(*
xml 存n行，每行4个参数，bool-可用位vaild、bool-输出位状态、bool-正反向输出标记位、lreal-节点坐标
*)

FUNCTION_BLOCK FB_EL5131_MultiCycle
VAR CONSTANT
	{attribute 'displaymode':='hex'}
	cMaxCounterValue										: 	UDINT := 4294967295;
	{attribute 'hide'}
	cMaxNumOfOutputPreCycle									:	USINT := 8;	 
END_VAR
VAR_INPUT
	{attribute 'hide'} // 隐藏该变量
	nDistWindow												:	UINT := 5;// pulse
	stEl5131												:	REFERENCE TO ST_EL5131;
	bReset													:	BOOL;
	bExecute												:	BOOL;
	bSetRefPos												:	BOOL;
	rRefPos													:	LREAL; // 以参考轴位置(mm)进行初始化
	rScaleFactor      										: 	LREAL := 1; // 分子/分母		            						: 	BYTE := 2#1111_1111;
	{attribute 'displaymode':='bin'}
	OutputOption											:	BYTE := 2#0000_0001; // chn 1 output
	InputOption												:	ST_EL5131_Setting;
	pstEL5131_CamData										:	POINTER TO ST_EL5131_CamData;
	nSize													:	ULINT;
	cNum													:	UDINT;// 点总数 >0
END_VAR
VAR_IN_OUT
	nActNum													:	UDINT;// presistent 第 0 个开始
END_VAR
VAR_OUTPUT
	bBusy													:	BOOL;
	bDone													:	BOOL;
	bError													:	BOOL;
	nErrId													:	UDINT;
	{attribute 'hide'}
	sErr													:	STRING;
END_VAR
VAR
	{attribute 'hide'}
	{attribute 'displaymode':='hex'}
	tDCTIME64												:	ULINT;
	{attribute 'hide'}
	{attribute 'displaymode':='hex'}
	LastTimeStampsOutChn1X64								: 	ARRAY[1..8] OF ULINT;
	{attribute 'hide'}
	{attribute 'displaymode':='hex'}
	LastTimeStampsOutChn2X64								: 	ARRAY[1..8] OF ULINT;
	{attribute 'hide'}
	_pLastTimeStampsOutChnX64								:	POINTER TO ARRAY[1..8] OF ULINT;
	{attribute 'hide'}
	{attribute 'displaymode':='hex'}
	TimeStampsOutChn1X64									: 	ARRAY[1..8] OF ULINT;
	{attribute 'hide'}
	{attribute 'displaymode':='hex'}
	TimeStampsOutChn2X64									: 	ARRAY[1..8] OF ULINT;
	{attribute 'hide'}
	{attribute 'displaymode':='hex'}
	_pTimestampChnX64										:	POINTER TO ARRAY[1..8] OF ULINT;// Point to stEl5131.PdoToPlc
	{attribute 'hide'}
	{attribute 'displaymode':='hex'}
	pPdoTimestampChnX32										:	POINTER TO ARRAY[1..8] OF ULINT;// Point to stEl5131.PdoToPlc
	{attribute 'hide'}
	rtReset                 								: 	R_TRIG;
	{attribute 'hide'}
	rtExecute                 								: 	R_TRIG;
	{attribute 'hide'}
	rtSetRefPos                								: 	R_TRIG;
	{attribute 'hide'}
	{attribute 'displaymode':='bin'}
	_nMem													:	WORD;// bit 0=reset ,bit 1=READY_TEMP load  
	{attribute 'hide'}
	_pControl												:	POINTER TO ST_Control_UINT_TO_BIT;
	{attribute 'hide'}
	_pControOutput											:	POINTER TO ST_ENC_Control_Output_Channel;
	{attribute 'hide'}
	i														:	INT;
	{attribute 'hide'}
	j														:	UDINT;
	eState													:	(INIT,LOAD,READY,RUN,FINISH);
	{attribute 'hide'}
	_tSetParDelay100ms										:	TON :=(PT:= T#0MS);
	{attribute 'hide'}
	_tSetParDelay5s											:	TON :=(PT:= T#5S);
	{attribute 'hide'}
	_tLastDurationDelay										:	TON :=(PT:= T#0S);
	
	{attribute 'hide'}
	_nTempLintComparDistWindow								:	LINT;
	{attribute 'hide'}
	_nLoadNum												:	UDINT;
	{attribute 'hide'}
	_cNum													:	UDINT;// 不足 8 个则按 8 个补全，因为 _pControOutput^.Number_of_output_events 不可在运行中改变
	{attribute 'hide'}
	_CamData												:	FB_MEM_TO_DATA_ST_EL5131_CamData;
	
END_VAR


rtReset(CLK:= bReset, Q=> );
IF rtReset.Q 
THEN 
	// reset
	A03_RESET();
ELSE
	// inti, set refpos
	rtSetRefPos(CLK:= bSetRefPos, Q=> );
	IF rtSetRefPos.Q 
	THEN
		_nMem.0												:= TRUE;// next step
		bBusy												:= TRUE;
		bDone												:= FALSE;
		bError												:= FALSE;
		nErrId												:= 0;
		sErr												:= '';
		_pControl											:= ADR(stEl5131.PlcToPdo.Control);
		IF _pControl^.Set_counter
		THEN 
			_pControl^.Set_counter							:= FALSE;// SetCounter
		END_IF
	ELSIF _nMem.0
	THEN
		_pControl											:= ADR(stEl5131.PlcToPdo.Control);
		stEl5131.PlcToPdo.Set_counter_value					:= TO_UDINT(rRefPos / rScaleFactor) MOD cMaxCounterValue;
		_tSetParDelay100ms(IN:= TRUE);
		IF _tSetParDelay100ms.Q // 0ms
		THEN 
			// set refpos
			A05_SetRefpos();
		END_IF	
	ELSE
		// work
		A04_WORK();
	END_IF
	
END_IF

ACTION A01_INIT:

// Contro_OutputChn1/2 cyclic
_pControOutput 												:= ADR(stEl5131.PlcToPdo.Contro_OutputChn1);
_pControOutput^.Control.Set_digital_output 					:= InputOption.SetDigitalOutput;
//_pControOutput^.Control.Enable_thresholds_output			:= InputOption.EnableThresholdsOutput;
_pControOutput^.Control.Set_tristate 						:= InputOption.SetTristate;
_pControOutput^.Control.Disalbe_thresholds_cw 				:= InputOption.DisableThresholdsCw;
_pControOutput^.Control.Disalbe_thresholds_ccw 				:= InputOption.DisableThresholdsCcw;
_pControOutput^.Number_of_output_events						:= cMaxNumOfOutputPreCycle;// _cNum 声明时有解释，按8的倍数补全

_pControOutput 												:= ADR(stEl5131.PlcToPdo.Contro_OutputChn2);
_pControOutput^.Control.Set_digital_output 					:= InputOption.SetDigitalOutput;
//_pControOutput^.Control.Enable_thresholds_output			:= InputOption.EnableThresholdsOutput;
_pControOutput^.Control.Set_tristate 						:= InputOption.SetTristate;
_pControOutput^.Control.Disalbe_thresholds_cw 				:= InputOption.DisableThresholdsCw;
_pControOutput^.Control.Disalbe_thresholds_ccw 				:= InputOption.DisableThresholdsCcw;
_pControOutput^.Number_of_output_events						:= cMaxNumOfOutputPreCycle;


_nMem														:= 0;
_nLoadNum													:= nActNum + 1;// eg:执行1个，重启后(nActNum=1)，从第2个开始
_cNum														:= SEL(cNum MOD cMaxNumOfOutputPreCycle = 0,(cNum / cMaxNumOfOutputPreCycle + 1)*cMaxNumOfOutputPreCycle,cNum);
IF OutputOption.0 
THEN // Contro_OutputChn1 TimestampChn1 LastTimeStampsOutChn1X64
	_pControOutput 											:= ADR(stEl5131.PlcToPdo.Contro_OutputChn1);
	pPdoTimestampChnX32										:= ADR(stEl5131.PdoToPlc.TimestampChn1);
	_pTimestampChnX64										:= ADR(TimeStampsOutChn1X64);
	_pLastTimeStampsOutChnX64								:= ADR(LastTimeStampsOutChn1X64);
END_IF
IF NOT OutputOption.0 
AND OutputOption.1
THEN // Contro_OutputChn2 TimestampChn2 LastTimeStampsOutChn2X64
	_pControOutput 											:= ADR(stEl5131.PlcToPdo.Contro_OutputChn2);
	pPdoTimestampChnX32										:= ADR(stEl5131.PdoToPlc.TimestampChn2);
	_pTimestampChnX64										:= ADR(TimeStampsOutChn2X64);
	_pLastTimeStampsOutChnX64								:= ADR(LastTimeStampsOutChn2X64);
END_IF
_pControOutput^.Output_state								:= 0;// 初始化 PDO_Output_state
_pControOutput^.Control.Enable_thresholds_output 			:= FALSE;// 复位时间戳
MEMSET(ADR(LastTimeStampsOutChn1X64),0,SIZEOF(LastTimeStampsOutChn1X64));
MEMSET(ADR(LastTimeStampsOutChn2X64),0,SIZEOF(LastTimeStampsOutChn2X64));
END_ACTION

ACTION A02_LAOD:


//FOR i:=1 TO cMaxNumOfOutputPreCycle BY 1
//DO
IF _nLoadNum <= _cNum
THEN 
	IF _nLoadNum > cNum // 处理超 arData[] 边界
	THEN
		;
		// _pControOutput^.Output_state._nIndex := pstEL5131_CamData^.arData[nActNum].bOutputState;
		_pControOutput^.Output_state						:= TO_USINT(CSETBIT32(_pControOutput^.Output_state,
																	TO_SINT(i-1),_CamData.get_bOutputState(cNum,pstEL5131_CamData)));
		IF _CamData.get_bBackward(cNum,pstEL5131_CamData) 
		THEN 
			;// 备用 cNum 最后一个元素
		ELSE 
			;
		END_IF
		// MOD cMaxCounterValue 溢出时直接取余，因为是单向触发，后32bit编码器值已满足
		_pControOutput^.Threshold[i]						:= TO_UDINT(_CamData.get_rPos(cNum,pstEL5131_CamData) / rScaleFactor) MOD cMaxCounterValue;
		_pControOutput^.Duration[i]							:= _CamData.get_nDuration(cNum,pstEL5131_CamData);
		_nLoadNum											:= _nLoadNum + 1;
	ELSE
		FOR j:=_nLoadNum TO cNum BY 1
		DO
			IF _CamData.get_bVaild(j,pstEL5131_CamData)
			THEN 
				// _pControOutput^.Output_state._nIndex := pstEL5131_CamData^.arData[nActNum].bOutputState;
				_pControOutput^.Output_state				:= TO_USINT(CSETBIT32(_pControOutput^.Output_state,
																	TO_SINT(i-1),_CamData.get_bOutputState(j,pstEL5131_CamData)));
				IF _CamData.get_bBackward(j,pstEL5131_CamData) 
				THEN 
					;// 备用 i-1
				ELSE 
					;
				END_IF
				_pControOutput^.Threshold[i]				:= TO_UDINT(_CamData.get_rPos(j,pstEL5131_CamData) / rScaleFactor) MOD cMaxCounterValue;
				_pControOutput^.Duration[i]					:= _CamData.get_nDuration(j,pstEL5131_CamData);
				_nLoadNum									:= _nLoadNum + 1;
				EXIT;// 寻到下一个 bVaild 则跳出 for(j) 循环
			END_IF		
		END_FOR	
	END_IF

END_IF
//END_FOR
END_ACTION

ACTION A03_RESET:
	bBusy 													:= FALSE;
	bDone													:= FALSE;
	bError													:= FALSE;
	nErrId													:= 0;
	sErr													:= '';
	eState 													:=	INIT;
	_nMem													:= 0;
	_nLoadNum												:= 1;
	nActNum													:= 0;
	_cNum													:= 0;
	_pControOutput 											:= ADR(stEl5131.PlcToPdo.Contro_OutputChn1);
	_pControOutput^.Control.Set_digital_output				:= FALSE;// set digital output
	_pControOutput^.Control.Set_tristate					:= FALSE;// set tristate
	_pControOutput^.Control.Enable_thresholds_output 		:= FALSE;// 复位时间戳
	_pControOutput 											:= ADR(stEl5131.PlcToPdo.Contro_OutputChn2);
	_pControOutput^.Control.Set_digital_output				:= FALSE;// set digital output
	_pControOutput^.Control.Set_tristate					:= FALSE;// set tristate
	_pControOutput^.Control.Enable_thresholds_output 		:= FALSE;// 复位时间戳
	_tSetParDelay100ms(IN:= FALSE);
	_tSetParDelay5s(IN:= FALSE);
END_ACTION

ACTION A04_WORK:
rtExecute(CLK:= bExecute, Q=> );
CASE eState OF 
	INIT:
		IF rtExecute.Q
		THEN 
			A01_Init();
			bBusy									:= TRUE;
			bDone									:= FALSE;
			bError									:= FALSE;
			nErrId									:= 0;
			sErr									:= '';
			IF pstEL5131_CamData = 0 OR rScaleFactor <= 0 OR cNum <= 0
			OR cNum > nSize / 16 // ST_EL5131_CamData 's size is 16
			THEN 
				bBusy								:= FALSE;
				bDone								:= FALSE;
				bError								:= TRUE;
				nErrId.1							:= TRUE;
				sErr								:= 'Param is not vaild';
			ELSE
				eState								:= LOAD;
			END_IF
		END_IF
	LOAD:
		IF nActNum >= _cNum // 初始化时，若 nActNum = _cNum ,也属于超范围
		OR nActNum < 0
		THEN 
			bBusy									:= FALSE;
			bDone									:= FALSE;
			bError									:= TRUE;
			nErrId.2								:= TRUE;
			sErr									:= 'nActNum out of range';
			eState									:= INIT;
		ELSIF nActNum < _cNum
		THEN
			FOR i:=1 TO cMaxNumOfOutputPreCycle BY 1
			DO
				A02_LAOD();// frist time
			END_FOR
			eState									:= READY;
			_pControOutput^.Control.Enable_thresholds_output := TRUE;
		END_IF
	READY:
		// Enable_thresholds_output := TRUE 时，时间戳 TimestampChn1 会变化，PDO 交互需要时间
		_nMem.1										:= TRUE;
		FOR i:=1 TO cMaxNumOfOutputPreCycle BY 1
		DO
			_pTimestampChnX64^[i]					:= pPdoTimestampChnX32^[i];
			IF _pTimestampChnX64^[i] <> _pLastTimeStampsOutChnX64^[i]
			AND _pTimestampChnX64^[i] <> 0 // init 使 _pLastTimeStampsOutChnX64^[i]=0,故要排除=0的情况
			THEN
				_pLastTimeStampsOutChnX64^[i]		:= _pTimestampChnX64^[i];
			END_IF
			_nMem.1									:= _nMem.1 AND _pTimestampChnX64^[i] = _pLastTimeStampsOutChnX64^[i]
														 	  AND _pTimestampChnX64^[i] <> 0;
		END_FOR
		IF _nMem.1
		THEN
			eState									:= RUN;
		END_IF
	RUN:
		IF nActNum > _cNum
		OR nActNum < 0
		THEN 
			bBusy									:= FALSE;
			bDone									:= FALSE;
			bError									:= TRUE;
			nErrId.2								:= TRUE;
			sErr									:= 'nActNum out of range';
			eState									:= INIT;
		ELSIF nActNum < _cNum
		THEN
			FOR i:=1 TO cMaxNumOfOutputPreCycle BY 1
			DO
				_pTimestampChnX64^[i]				:= pPdoTimestampChnX32^[i];
				IF _pTimestampChnX64^[i] <> _pLastTimeStampsOutChnX64^[i]
				THEN
					_pLastTimeStampsOutChnX64^[i]	:= _pTimestampChnX64^[i];
					A02_LAOD();// cyclic
					nActNum 						:= nActNum + 1;
				END_IF
			END_FOR
		ELSE // nActNum = _cNum
			IF _pControOutput^.Duration[8] <> 0 // 等待最后一个延时到达
			THEN
				_tLastDurationDelay(IN:= TRUE,PT:= TO_TIME(_pControOutput^.Duration[8])/1000);// to_time unit=ms,Duration's unit=us
				IF _tLastDurationDelay.Q
				THEN// done
					bBusy							:= FALSE;
					bDone							:= TRUE;
					bError							:= FALSE;
					nErrId							:= 0;
					sErr							:= '';
					eState							:= INIT;
					_pControOutput 					:= ADR(stEl5131.PlcToPdo.Contro_OutputChn1);
					_pControOutput^.Control.Enable_thresholds_output := FALSE;
					_pControOutput 					:= ADR(stEl5131.PlcToPdo.Contro_OutputChn2);
					_pControOutput^.Control.Enable_thresholds_output := FALSE;	
					_tLastDurationDelay(IN:= FALSE);
				END_IF
			ELSE// done
				bBusy								:= FALSE;
				bDone								:= TRUE;
				bError								:= FALSE;
				nErrId								:= 0;
				sErr								:= '';
				eState								:= INIT;
				_pControOutput 						:= ADR(stEl5131.PlcToPdo.Contro_OutputChn1);
				_pControOutput^.Control.Enable_thresholds_output := FALSE;
				_pControOutput 						:= ADR(stEl5131.PlcToPdo.Contro_OutputChn2);
				_pControOutput^.Control.Enable_thresholds_output := FALSE;	
				_tLastDurationDelay(IN:= FALSE);
			END_IF
			
		END_IF
END_CASE
END_ACTION

ACTION A05_SetRefpos:
_pControl^.Set_counter							:= TRUE;
_tSetParDelay5s(IN:= TRUE);
IF stEl5131.PdoToPlc.Status.Set_counter_done 
THEN 
	_nTempLintComparDistWindow					:= ABS(TO_LINT(stEl5131.PdoToPlc.Counter_value)
													 - TO_LINT(stEl5131.PlcToPdo.Set_counter_value));
	IF  _nTempLintComparDistWindow <= nDistWindow
	THEN 
		_pControl^.Set_counter					:= FALSE;
		bBusy									:= FALSE;
		bError									:= FALSE;
		bDone									:= TRUE;
		nErrId									:= 0;
		sErr									:= '';
		_nMem.0									:= FALSE;// next step
		_tSetParDelay100ms(IN:= FALSE);
		_tSetParDelay5s(IN:= FALSE);
	END_IF
ELSIF _tSetParDelay5s.Q
THEN 
	_pControl^.Set_counter						:= FALSE;
	bBusy										:= FALSE;
	bDone										:= FALSE;
	bError										:= TRUE;
	nErrId.0									:= TRUE;
	sErr										:= 'EL5151 SetPos | SetVal <> ActVal';
	_nMem.0										:= FALSE;
	_tSetParDelay100ms(IN:= FALSE);
	_tSetParDelay5s(IN:= FALSE);
END_IF
END_ACTION

END_FUNCTION_BLOCK
